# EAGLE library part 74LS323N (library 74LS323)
74LS323
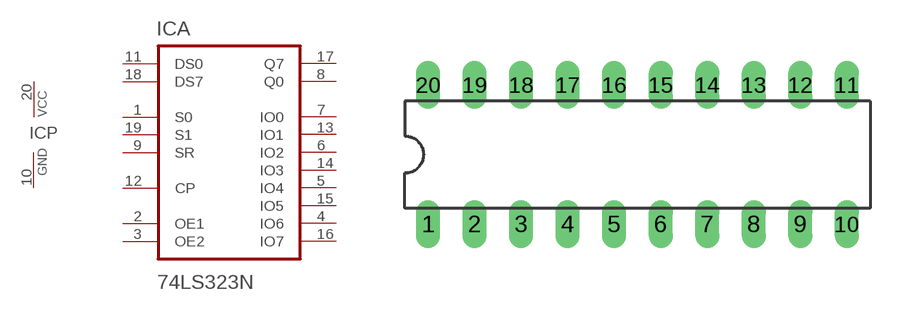
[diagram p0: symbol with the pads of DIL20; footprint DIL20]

Designator prefix IC; gates A=74LS323N P=PWRN

## 74LS323N  [DIL20]
1  A:S0  in
2  A:OE1  in
3  A:OE2  in
4  A:IO6  out
5  A:IO4  out
6  A:IO2  out
7  A:IO0  out
8  A:Q0  in
9  A:SR  in
10  P:GND  pwr
11  A:DS0  in
12  A:CP  in
13  A:IO1  out
14  A:IO3  out
15  A:IO5  out
16  A:IO7  out
17  A:Q7  in
18  A:DS7  in
19  A:S1  in
20  P:VCC  pwr

## Footprint DIL20 (pad centres in mm)
Dual In Line Package
drill 0.813 long: 1 -8.89,-3.81; 2 -6.35,-3.81; 3 -3.81,-3.81; 4 -1.27,-3.81; 5 1.27,-3.81; 6 3.81,-3.81; 7 6.35,-3.81; 8 8.89,-3.81; 9 11.43,-3.81; 10 13.97,-3.81; 11 13.97,3.81; 12 11.43,3.81; 13 8.89,3.81; 14 6.35,3.81; 15 3.81,3.81; 16 1.27,3.81; 17 -1.27,3.81; 18 -3.81,3.81; 19 -6.35,3.81; 20 -8.89,3.81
